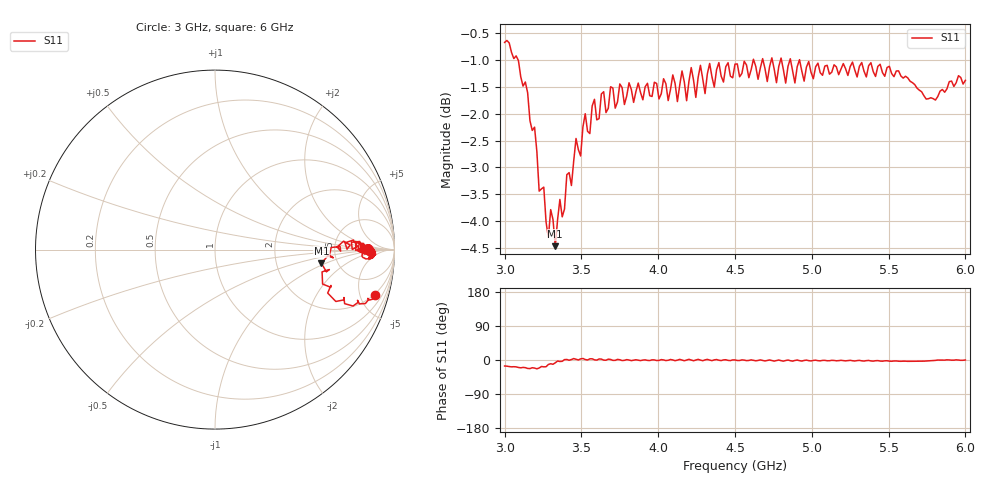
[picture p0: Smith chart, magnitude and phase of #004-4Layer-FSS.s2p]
!  05/08/2025  16:27:08
! Ref Plane: 0.000 mm
# MHZ S MA R  50
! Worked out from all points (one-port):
!   201 points, 3 GHz to 6 GHz, reference 50 ohm
!   lowest |S11| = -4.5 dB at 3.33 GHz (marker M1), VSWR 3.98, Z = 187 - j44.7 ohm
!   |S11| at or under -10 dB: nowhere
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3000  0.9254 -15.8
3135  0.8501 -20.2
3210  0.7325 -23.2
3330  0.598 -7.4
3375  0.6368 -3.5
3450  0.7179 3.8
3525  0.7943 1.3
3555  0.7612 3.1
3585  0.8191 0.5
3750  0.8466 0.7
4065  0.817 -0.7
4095  0.8631 0.1
4125  0.8152 -0.3
4155  0.8705 0.0
4185  0.8168 -0.2
4215  0.8768 -0.1
4245  0.8225 0.0
4275  0.8811 -0.2
4305  0.8293 0.3
4335  0.8846 -0.2
4365  0.8409 0.3
4500  0.8834 0.1
4845  0.8791 -0.1
4875  0.8711 -3.0
4905  0.8785 -0.1
5250  0.8787 -0.8
5625  0.8576 -3.5
6000  0.8532 0.0
